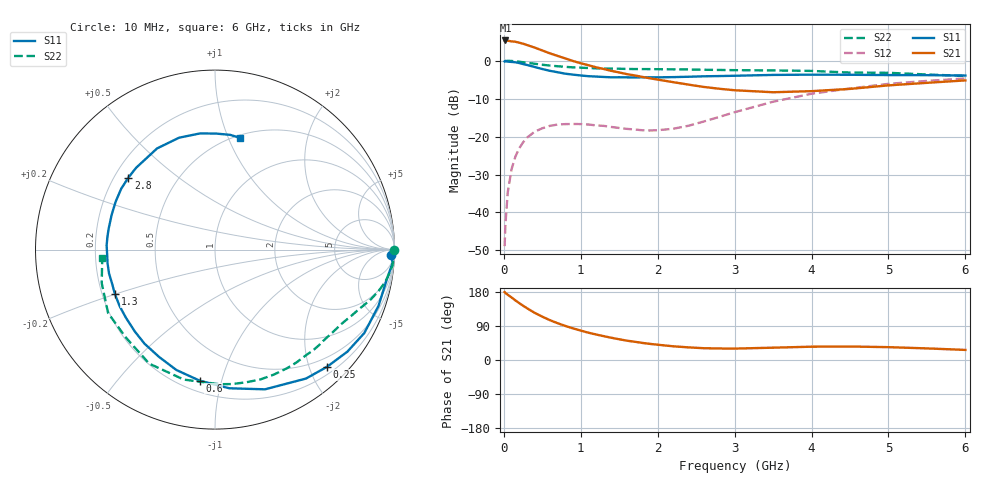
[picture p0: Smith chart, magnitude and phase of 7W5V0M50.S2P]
! Infineon Technologies  Discrete & RF Semiconductors
! BFS17W
! Si NPN RF Bipolar Junction Transistor in SOT323
! VCE = 5 V  IC = 0.5 mA
! Common Emitter S-Parameters:  August  1999
# GHz  S  MA  R  50
!  f  S11  S21  S12  S22
! GHz  MAG  ANG  MAG  ANG  MAG  ANG  MAG  ANG
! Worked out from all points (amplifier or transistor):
!   36 points, 10 MHz to 6 GHz, reference 50 ohm
!   highest |S21| = 5.3 dB at 20 MHz (marker M1)
!   |S21| within 3 dB of that: start of sweep to 547.4 MHz
!   unconditionally stable (mu >= 1): 1.224 GHz to end of sweep
!   at 250 MHz: K = 0.22, MSG = 13.0 dB, |S12| = -21.5 dB
!   at 1.4 GHz: K = 1.14, MAG = 5.1 dB, |S12| = -17.5 dB
!   at 6 GHz: K = 1.09, MAG = -2.1 dB, |S12| = -4.7 dB
!   S11 on the Smith chart (normalised r, x): 10 MHz: 30, -43; 250 MHz: 0.32, -2.30; 600 MHz: 0.27, -0.85; 1.3 GHz: 0.25, -0.20; 2.8 GHz: 0.26, +0.34; 6 GHz: 0.53, +1.11
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0.01  0.9784 -1.8  1.834 179.3  0.0036 87.6  0.9999 0.0
0.02  0.993 -4.1  1.848 177.1  0.0067 95.1  0.9868 -1.0
0.05  0.9719 -9.7  1.836 172.3  0.0182 85.6  0.9966 -2.6
0.1  0.9634 -19.0  1.797 165.1  0.0371 78.4  0.992 -5.3
0.15  0.9529 -29.2  1.777 157.3  0.0545 72.9  0.9805 -7.7
0.25  0.9033 -46.3  1.675 143.3  0.0839 62.3  0.9547 -12.2
0.3  0.8793 -54.8  1.61 136.8  0.0966 57.9  0.9408 -14.1
0.4  0.8268 -70.3  1.489 124.6  0.116 50.0  0.9114 -17.7
0.5  0.7768 -84.1  1.364 114.3  0.1287 43.3  0.8843 -20.6
0.6  0.7351 -96.7  1.249 105.0  0.1386 38.0  0.8627 -23.2
0.8  0.6741 -117.6  1.07 89.9  0.1461 30.5  0.8295 -28.2
1.1  0.6249 -142.5  0.872 72.0  0.1442 24.5  0.8007 -35.3
1.3  0.6102 -156.0  0.777 62.8  0.1383 23.5  0.7887 -40.3
1.6  0.6035 -172.8  0.665 51.0  0.1264 26.9  0.7789 -48.0
2.2  0.6076 161.4  0.522 36.2  0.1268 48.6  0.7698 -64.7
2.8  0.6275 140.3  0.427 30.4  0.1817 65.4  0.7553 -82.7
3.5  0.6496 119.8  0.384 32.5  0.2881 66.3  0.7448 -103.5
4  0.6548 107.8  0.397 35.1  0.3669 60.6  0.7335 -120.0
4.5  0.6526 97.4  0.425 35.6  0.4308 53.4  0.6975 -135.5
5  0.6466 89.5  0.473 33.9  0.4955 46.3  0.6927 -149.3
5.5  0.6448 82.5  0.511 30.6  0.5418 39.2  0.6582 -163.5
6  0.6379 77.2  0.55 26.6  0.5836 32.7  0.6299 -175.9
